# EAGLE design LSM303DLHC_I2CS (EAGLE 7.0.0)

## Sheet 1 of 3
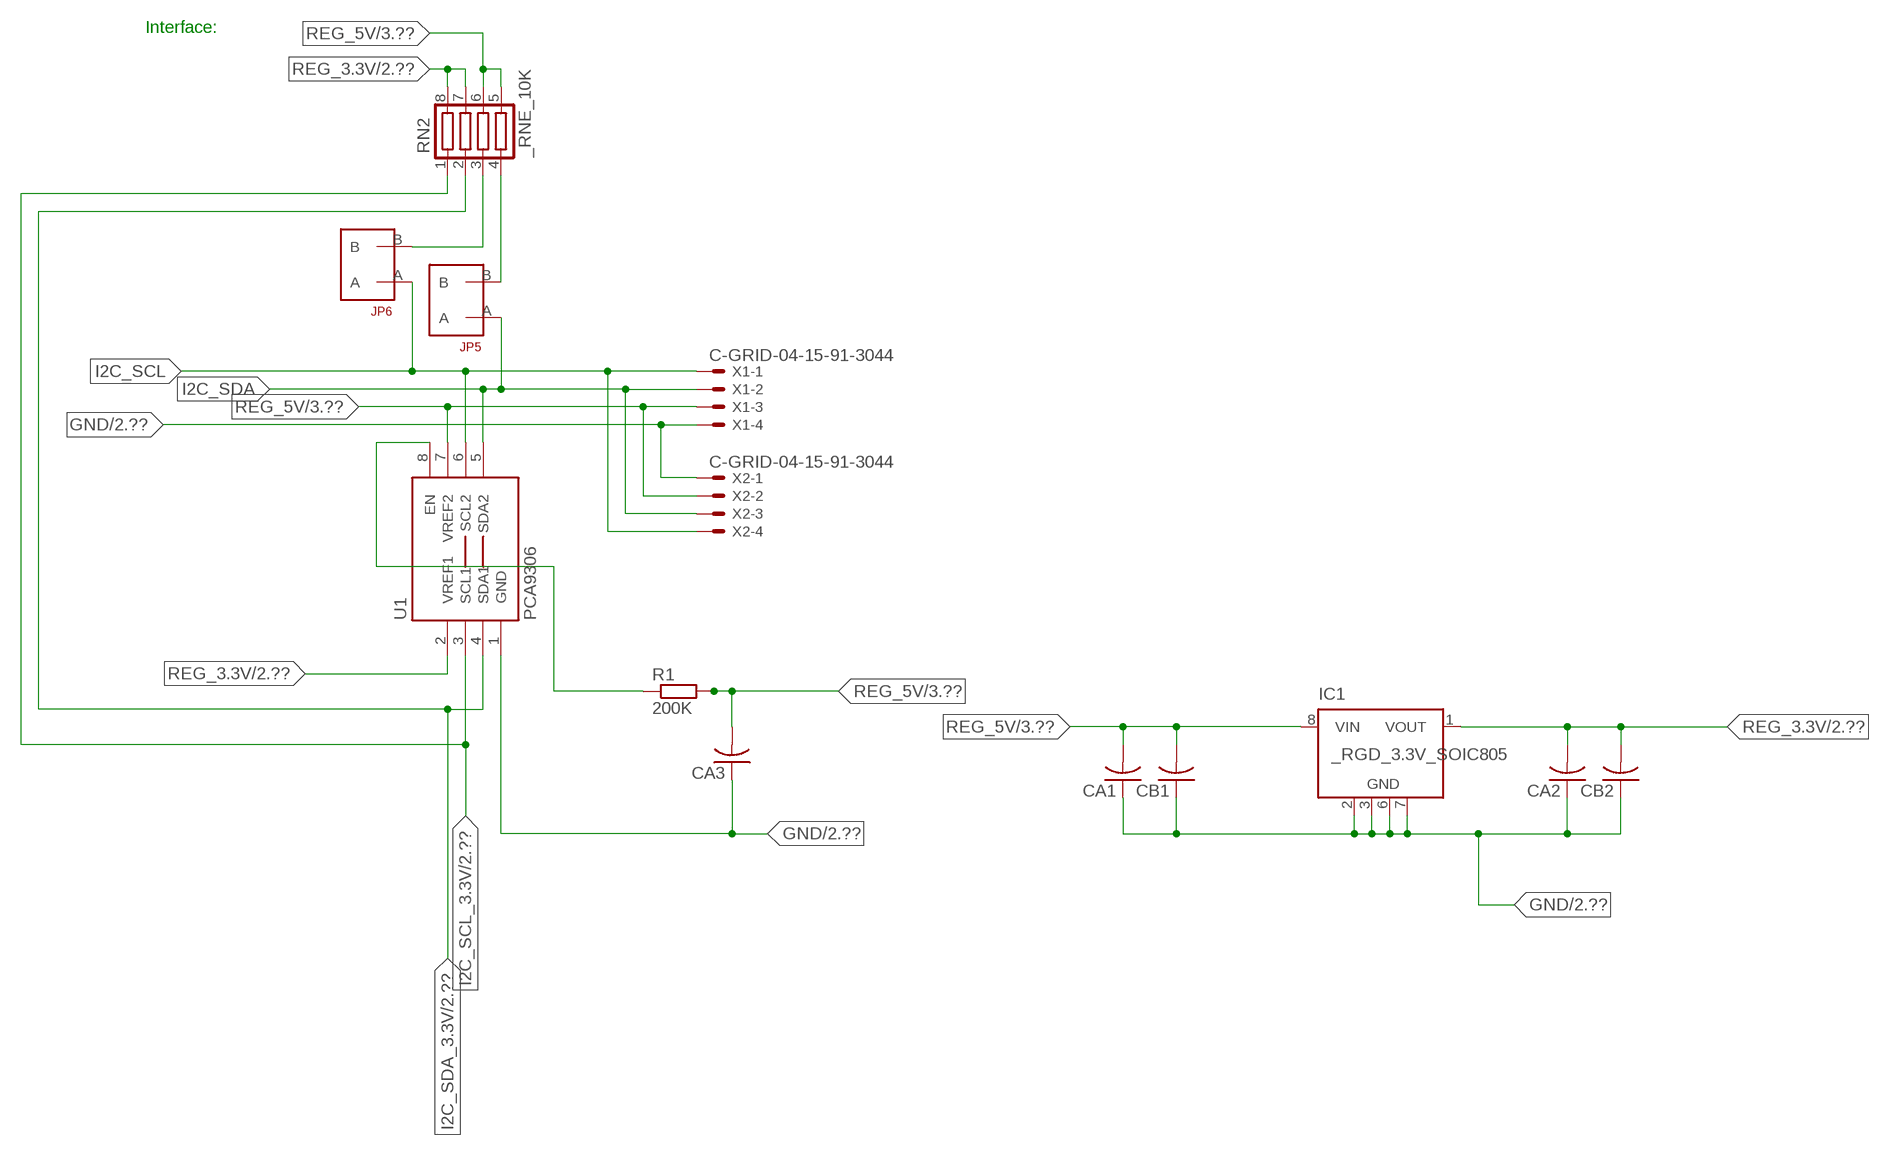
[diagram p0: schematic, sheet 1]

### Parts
CA1  CC1206KRX7R9BB104  [.1UF]
CA2  CC1206KRX7R9BB104  [.1UF]
CA3  CC1206KRX7R9BB104  [.1UF]
CB1  TMK316F106ZL-TC1206K  [TMK316F106ZL-T]
CB2  TMK316F106ZL-TC1206K  [TMK316F106ZL-T]
IC1  _RGD_3.3V_SOIC805  [_RGC_3.3V_SOIC8]
JP5  JUMPER_1X2_2MM  [JUMPER_1X2_2MM]
JP6  JUMPER_1X2_2MM  [JUMPER_1X2_2MM]
R1  200K  RESISTOR_SMT-0603  [R603]
RN2  _RNE_10K  [RNE]
U1  PCA9306  PCA9306_NCD  [PSOP-8]
X1  C-GRID-04-15-91-3044  [15-91-04]
X2  C-GRID-04-15-91-3044  [15-91-04]

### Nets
GND: CA1.1 CA2.1 CA3.1 CB1.1 CB2.1 IC1.2(GND) IC1.3(GND) IC1.6(GND) IC1.7(GND) U1.1(GND) X1.4 X2.1 ; also sheet 2,3
I2C_SCL: JP6.A U1.6(SCL2) X1.1 X2.4
I2C_SCL_3.3V: RN2.1 U1.3(SCL1) ; also sheet 2
I2C_SDA: JP5.A U1.5(SDA2) X1.2 X2.3
I2C_SDA_3.3V: RN2.2 U1.4(SDA1) ; also sheet 2
N$1: JP6.B RN2.3
N$2: JP5.B RN2.4
N$3: R1.1 U1.8(EN)
REG_3.3V: CA2.2 CB2.2 IC1.1(VOUT) RN2.7 RN2.8 U1.2(VREF1) ; also sheet 2
REG_5V: CA1.2 CA3.2 CB1.2 IC1.8(VIN) R1.2 RN2.5 RN2.6 U1.7(VREF2) X1.3 X2.2 ; also sheet 3
Unconnected: IC1.4(NC) IC1.5(NC)

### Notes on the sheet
- Interface:

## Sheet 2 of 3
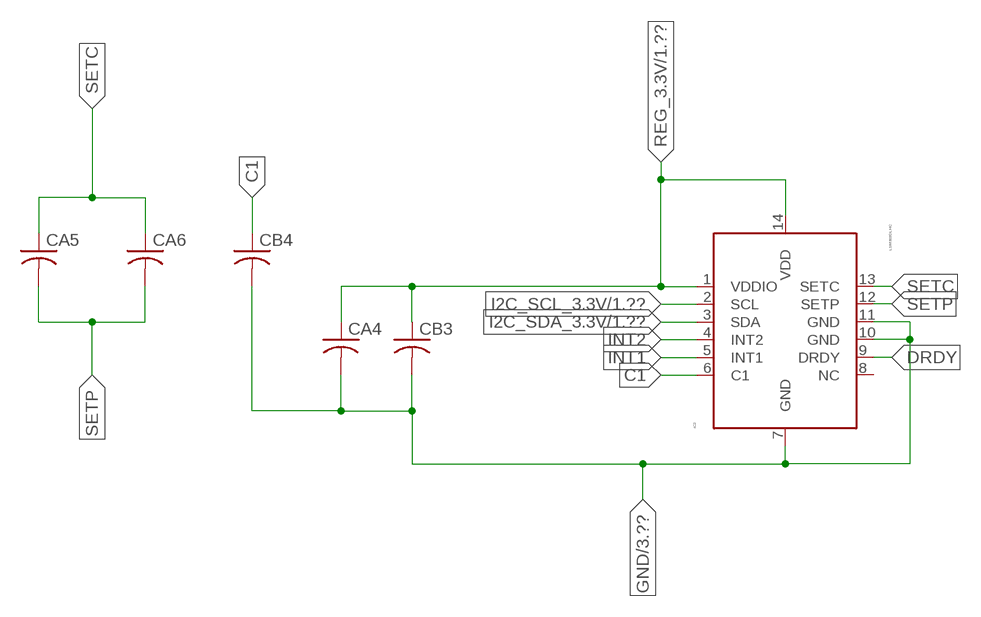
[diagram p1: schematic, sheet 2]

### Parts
CA4  CC1206KRX7R9BB104  [.1UF]
CA5  CC1206KRX7R9BB104  [.1UF]
CA6  CC1206KRX7R9BB104  [.1UF]
CB3  _CB_10UF_25VC1206K  [_CB_10UF_25V]
CB4  _CB_10UF_25VC1206K  [_CB_10UF_25V]
IC2  LSM303DLHC  MICROBUILDER_LSM303DLHC  [MICROBUILDER_LGA14]

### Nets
C1: CB4.1 IC2.6(C1)
DRDY: IC2.9(DRDY)
GND: CA4.2 CB3.2 CB4.2 IC2.7(GND) IC2.10(GND) IC2.11(GND) ; also sheet 1,3
I2C_SCL_3.3V: IC2.2(SCL) ; also sheet 1
I2C_SDA_3.3V: IC2.3(SDA) ; also sheet 1
INT1: IC2.5(INT1)
INT2: IC2.4(INT2)
REG_3.3V: CA4.1 CB3.1 IC2.1(VDDIO) IC2.14(VDD) ; also sheet 1
SETC: CA5.1 CA6.1 IC2.13(SETC)
SETP: CA5.2 CA6.2 IC2.12(SETP)
Unconnected: IC2.8(NC)

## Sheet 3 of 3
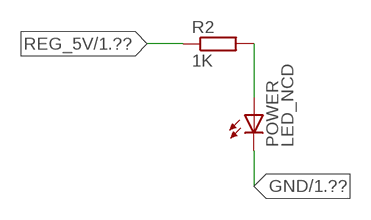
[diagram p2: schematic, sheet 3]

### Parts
POWER  LED_NCD  [CHIPLED_0603]
R2  1K  RESISTOR_SMT-0402  [R402]

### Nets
GND: POWER.C ; also sheet 1,2
N$4: POWER.A R2.2
REG_5V: R2.1 ; also sheet 1

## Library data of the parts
CA1-CA3 = NCD_ULTIMATE_LIBRARY:CC1206KRX7R9BB104: Capacitor CA .1uF 50V SMT C1206K CC1206KRX7R9BB104
CA4-CA6 = NCD_ULTIMATE_LIBRARY (2):CC1206KRX7R9BB104: Capacitor CA .1uF 50V SMT C1206K CC1206KRX7R9BB104
CB1 CB2 = NCD_ULTIMATE_LIBRARY:TMK316F106ZL-T: Capacitor CB 10uF SMT 1206 TMK316F106ZL-T
CB3 CB4 = NCD_ULTIMATE_LIBRARY (2):_CB_10UF_25V: Capacitor 10uF SMT
IC1 = NCD_ULTIMATE_LIBRARY:_RGD_3.3V_SOIC8: Regulator Linear 3.3V Chip Positive VOLTAGE REGULATOR Digikey 497-1199-2-ND/L78L33ACD13TR
IC2 = NCD_ULTIMATE_KAMNA:MICROBUILDER_LSM303DLHC: LSM303DLHC 3-Axis I2C Accelerometer and 3-Axis Magnetometer VDD: 2.2-3.6V VDDIO: 1.8-VDD Magnetic Range: +/-1.3 to +/-8.1 gauss Accel Range: +/-2/4/8/16 g Temp: -40 - 85°C
JP5 JP6 = NCD_ULTIMATE_CONNECTORS:JUMPER_1X2_2MM
POWER = NCD_ULTIMATE_LIBRARY:LED_NCD: LED Digikey 754-1132-2-ND/APT2012SRCPRV
R1 R2 = NCD_ULTIMATE_LIBRARY:RESISTOR_SMT: NCD Resistor
RN2 = NCD_ULTIMATE_LIBRARY:_RNE_10K: Resistor Array RNE SMT 10K x 4 Single Resistor Source: http://www.ctscorp.com/components/Datasheets/CTSChipArrayDs.pdf Digikey 742C083103JPTR-ND/742C083103JP; OC_FARNELL: unknown; OC_NEWARK: unknown
U1 = NCD_ULTIMATE_LIBRARY:PCA9306_NCD: NCD Bidirectional I2C level shifter. NOT compatible with all available part number pinout schemes- DOUBLE CHECK!!!; PROD_ID: IC-10023
X1 X2 = NCD_ULTIMATE_CONNECTORS:C-GRID-04: CONNECTOR 4-Pos I2C wire to board 2.54 mm (0.100") pitch header Digikey WM1342-ND/0015912045; OC_FARNELL: unknown; OC_NEWARK: unknown

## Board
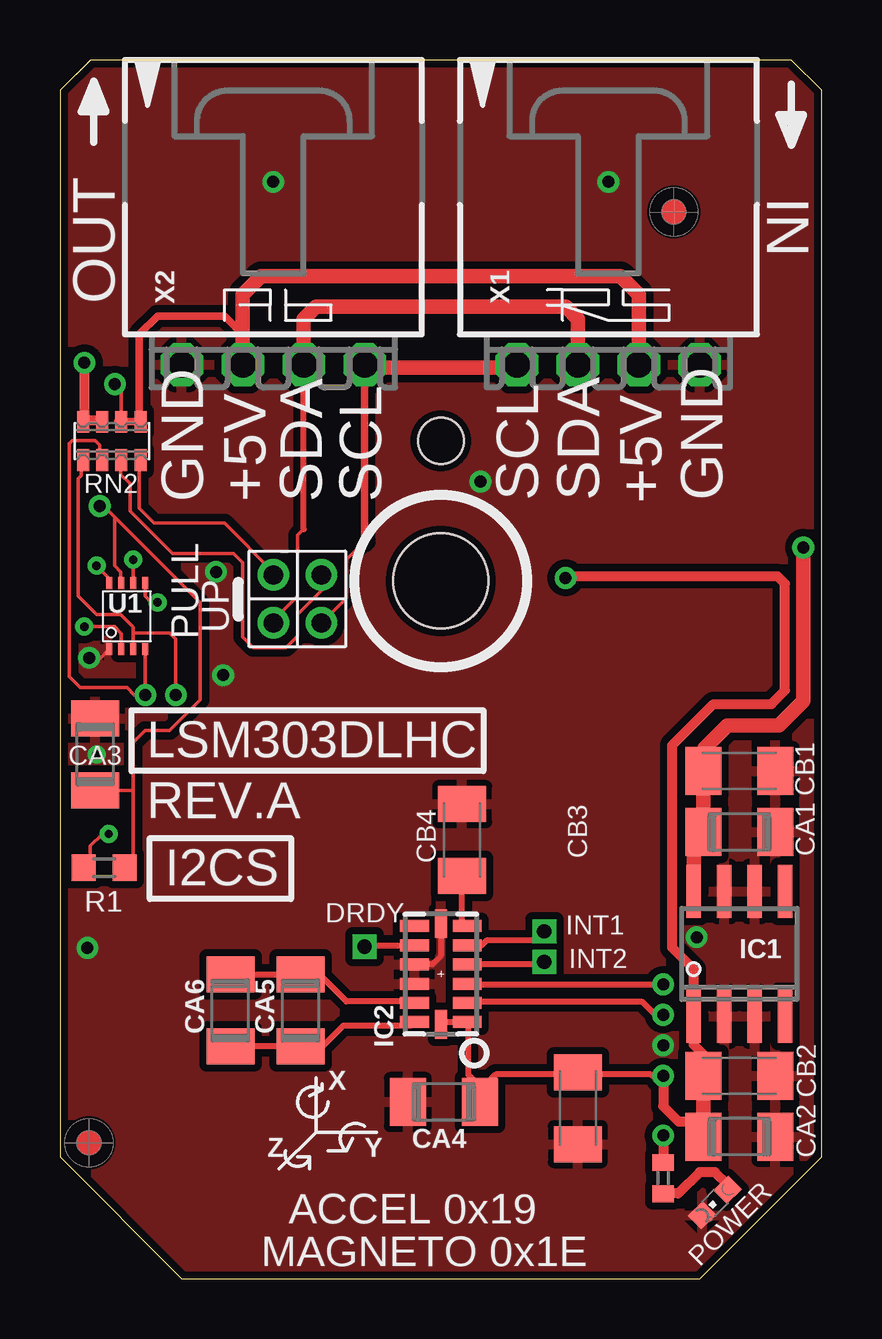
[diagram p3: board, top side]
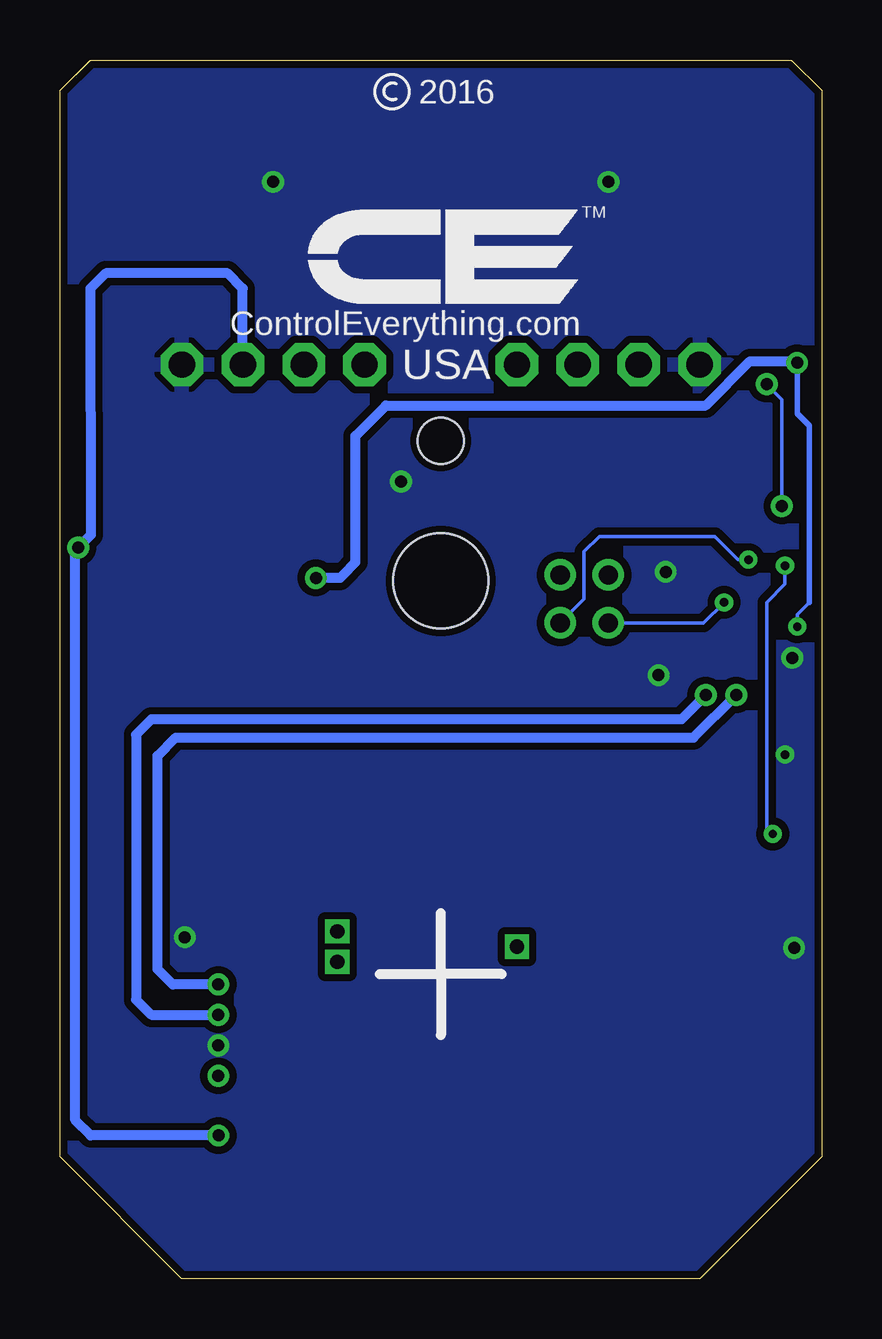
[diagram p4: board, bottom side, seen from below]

Size 31.75 x 50.8 mm. Coordinates in mm from the lower left corner, seen from the top.
Outline: 32 segments
Copper layers (1*16): Top 0.035mm / dielectric 1.5mm / Bottom 0.035mm
Design rules "default": minimum track width 5mil, minimum drill 24mil, track to track 5mil, track to pad 5mil, pad to pad 5mil, via to via 5mil, smd to smd 5mil, copper to edge 10mil, drill to drill 8mil, minimum pad ring 10mil, minimum via ring 8mil, stop-mask expansion 2mil, vias tented up to drill 0mil, thermal gap 10mil
Holes 3.96 mm at 15.88,29.08
Holes 1.91 mm at 15.88,34.93

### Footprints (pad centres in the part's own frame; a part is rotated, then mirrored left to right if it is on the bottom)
.1UF = smd 1.5 x 2: 1 -1.5,0; 2 1.5,0
TMK316F106ZL-T = smd 1.5 x 2: 1 -1.5,0; 2 1.5,0
_CB_10UF_25V = smd 1.5 x 2: 1 -1.5,0; 2 1.5,0
_RGC_3.3V_SOIC8 = smd 0.6 x 2.2: 1 -1.905,-2.6; 2 -0.635,-2.6; 3 0.635,-2.6; 4 1.905,-2.6; 5 1.905,2.6; 6 0.635,2.6; 7 -0.635,2.6; 8 -1.905,2.6
MICROBUILDER_LGA14 = smd 0.5 x 1.2: 1 2,1.1; 2 1.2,1.1; 3 0.4,1.1; 4 -0.4,1.1; 5 -1.2,1.1; 6 -2,1.1; 8 -2,-1.1; 9 -1.2,-1.1; 10 -0.4,-1.1; 11 0.4,-1.1; 12 1.2,-1.1; 13 2,-1.1 | smd 1.2 x 0.5: 7 -2.1,0; 14 2.1,0
JUMPER_1X2_2MM = drill 0.8: A 0,2; B 0,0
CHIPLED_0603 = smd 0.8 x 0.876: A 0,-0.75; C 0,0.75
R603 = smd 1 x 1.1: 1 -0.85,0; 2 0.85,0
R402 = smd 0.7 x 0.9: 1 -0.65,0; 2 0.65,0
RNE = smd 0.5 x 0.9: 1 -1.2,-0.8; 2 -0.4,-0.8; 3 0.4,-0.8; 4 1.2,-0.8; 5 1.2,0.8; 6 0.4,0.8; 7 -0.4,0.8; 8 -1.2,0.8
PSOP-8 = smd 0.25 x 0.5: 1 -0.73,-1.37; 2 -0.23,-1.37; 3 0.27,-1.37; 4 0.77,-1.37; 5 0.77,1.38; 6 0.27,1.38; 7 -0.23,1.38; 8 -0.73,1.38
15-91-04 = drill 1.1 pad 1.778 octagon: 1 -3.81,-7.62; 2 -1.27,-7.62; 3 1.27,-7.62; 4 3.81,-7.62

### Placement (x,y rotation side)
CA1  28.32,18.62 180 top
CA2  28.32,5.92 180 top
CA3  1.46,21.86 270 top
CA4  16,7.37 180 top
CA5  10.03,11.18 90 top
CA6  7.11,11.18 90 top
CB1  28.32,21.16 180 top
CB2  28.32,8.46 180 top
CB3  21.59,7.11 270 top
CB4  16.76,18.29 90 top
IC1  28.32,13.54 0 top
IC2  15.88,12.7 270 top
JP5  8.89,29.34 180 top
JP6  10.9,29.34 180 top
POWER  27.3,3.18 135 top
R1  1.84,17.13 0 top
R2  25.15,4.19 270 top
RN2  2.16,34.93 0 top
U1  2.79,27.61 0 top
U$5  [VISION_REF10]  1.21,5.66 90 top
U$28  [VISION_REF10]  25.59,44.46 90 top
X1  22.86,45.72 0 top
X2  8.89,45.72 0 top

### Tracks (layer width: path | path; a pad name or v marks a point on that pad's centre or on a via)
C1
  Top 0.254: IC2.6 16.76,14.91 CB4.1
DRDY  (via drill 0.6)
  Top 0.254: v12.7,13.84 12.76,13.9 IC2.9
GND  (via drill 0.35, 0.5)
  Top 0.152: CA3.1 1.52,23.42 1.52,23.62 | U1.1 1.7,25.88 v1.22,25.88
  Top 0.254: IC2.7 15.88,13.46 15.51,13.1 IC2.10
  other vias: 8.89,45.72 22.86,45.72 25.15,9.73 6.8,25.16 17.53,33.22 26.55,14.24 1.15,13.79 6.5,29.46 1.52,21.84
  pour Top (isolate 0.305): -1.27,0 -1.27,50.8 33.02,50.8 33.02,0
  pour Bottom (isolate 0.305): -5.08,0 -5.08,50.8 35.56,50.8 35.56,0
I2C_SCL  (via drill 0.35)
  Top 0.152: 12.7,30.73 11.94,29.97 11.94,28.38 JP6.A | v3.05,29.97 3.06,29.96 U1.6
  Top 0.305: 12.7,30.73 X2.4
  Top 0.406: X2.4 12.7,37.97 | 19.05,37.97 X1.1
  Top 0.61: 12.7,37.97 19.05,37.97
  Bottom 0.152: JP6.A 9.91,28.33 9.91,30.3 9.27,30.94 4.45,30.94 3.48,29.97 v3.05,29.97
I2C_SCL_3.3V  (via drill 0.5)
  Top 0.152: RN2.1 0.89,34.07 0.89,33.48 0.77,33.35 0.77,29.1 0.76,29.09 0.76,28.45 1.52,27.69 2.54,27.69 3.06,27.17 3.06,26.92 | 3.06,26.92 U1.3 | v4.83,24.33 v4.83,24.34 4.83,26.67 4.57,26.92 3.06,26.92
  Top 0.254: IC2.2 17.03,11.56 24.26,11.56 24.82,11 v25.15,11
  Bottom 0.406: v4.83,24.33 5.84,23.32 27.94,23.32 28.58,22.68 28.58,11.63 27.94,11 v25.15,11
I2C_SDA  (via drill 0.35)
  Top 0.152: JP5.A 8.89,27.44 9.91,28.45 9.91,30.99 10.16,31.24 | U1.5 3.56,28.45 3.81,28.19 v4.06,28.19
  Top 0.254: 10.16,31.24 10.16,31.25 X2.3
  Top 0.61: X2.3 10.16,40.01 10.67,40.51 21.09,40.51 21.59,40.01 X1.2
  Bottom 0.152: v4.06,28.19 4.92,27.34 JP5.A
I2C_SDA_3.3V  (via drill 0.5)
  Top 0.152: RN2.2 1.65,34.14 1.65,34.75 1.46,34.94 0.51,34.94 0.38,34.81 0.38,26.37 0.38,26.36 0.38,25.1 0.84,24.64 2.79,24.64 3.1,24.33 v3.56,24.33 v3.56,24.34 U1.4
  Top 0.254: IC2.3 17.01,12.27 v25.15,12.27
  Bottom 0.406: v25.15,12.27 27.05,12.27 27.69,12.9 27.69,21.79 26.93,22.56 5.34,22.56 v3.56,24.33
INT1  (via drill 0.6)
  Top 0.254: v20.19,14.48 19.81,14.1 17.78,14.1 17.58,13.9 IC2.5
INT2  (via drill 0.6)
  Top 0.254: v20.19,13.21 20.09,13.1 IC2.4
N$1
  Top 0.152: JP6.B 10.92,29.31 10.92,28.7 9.91,27.69 9.91,26.8 9.42,26.31 8.06,26.31 7.62,26.75 7.62,29.84 7.24,30.23 4.7,30.23 2.92,32 2.92,33.15 2.54,33.53 2.54,34.1 RN2.3
  Top 0.305: 2.54,34.02 RN2.3
N$2
  Top 0.152: JP5.B 8.89,29.46 6.86,31.5 3.94,31.5 3.3,32.13 3.3,34.07 RN2.4
  Top 0.305: 3.37,33.88 RN2.4
N$3  (via drill 0.35)
  Top 0.152: R1.1 1.27,17.41 1.27,18.03 1.78,18.54 v2.03,18.54 | v1.52,29.72 2.06,29.18 U1.8
  Bottom 0.152: v2.03,18.54 2.29,18.8 2.29,28.19 1.52,28.96 v1.52,29.72
N$4
  Top 0.406: POWER.A 27.84,3.92 27.3,4.45 26.67,4.45 25.78,3.56 25.16,3.56 R2.2
REG_3.3V  (via drill 0.35, 0.5)
  Top 0.152: v1.02,27.18 2.29,27.18 2.56,26.9 U1.2
  Top 0.254: IC2.14 15.97,10.7 IC2.1 | IC2.1 17.02,10.66 17.02,8.51 17.4,8.13 CA4.1 17.78,8.13 18.16,8.51 21.59,8.51 | IC2.1 17.01,10.67 | v25.15,8.46 24.69,8.46 24.64,8.51 21.59,8.51 | CB3.1 21.59,8.51
  Top 0.406: CB2.2 26.82,9.35 26.42,9.75 26.42,10.36 | v25.15,8.46 25.15,7.19 25.78,6.55 26.82,6.55 | IC1.1 26.42,12.9 25.53,13.79 25.53,22.24 27.24,23.95 29.66,23.95 30.23,24.52 30.23,28.97 29.91,29.29 21.16,29.29 v21.08,29.21 | 26.52,5.62 CA2.2 | v1.02,38.18 1.02,35.78 | 1.02,35.78 RN2.8 | 1.02,35.78 1.71,35.78 RN2.7
  Top 0.61: CB2.2 26.82,6.55 CA2.2 | 26.42,10.36 IC1.1
  Bottom 0.152: 0.51,28.19 1.02,27.69 v1.02,27.18
  Bottom 0.229: 0.51,28.19 0.51,35.56 1.02,36.07 v1.02,38.18
  Bottom 0.406: v1.02,38.18 1.08,38.24 2.99,38.24 4.83,36.4 18.16,36.4 19.43,35.13 19.43,29.87 19.94,29.34 20.07,29.21 v21.08,29.21
REG_5V  (via drill 0.5)
  Top 0.152: RN2.6 2.56,37.01 v2.29,37.29 | R1.2 3.05,17.49 3.05,20.36 | 3.05,20.36 3.05,22.35 3.56,22.86 4.57,22.86 5.84,24.13 5.84,28.19 2.29,31.75 | CA3.2 3.05,20.36 | 2.29,31.75 1.83,32.21 v1.65,32.21 | U1.7 2.54,29.01 2.54,29.46 2.29,29.72 2.29,31.75
  Top 0.305: 7.62,39.37 7.5,39.37 | 2.42,35.74 RN2.6 RN2.5 3.31,35.8 3.31,39.37 4.07,40.13 6.86,40.13 7.62,39.37 | X2.2 7.62,39.37
  Top 0.406: v25.15,5.97 R2.1
  Top 0.61: X2.2 7.62,41.02 8.38,41.78 23.37,41.78 24.13,41.02 X1.3 | IC1.8 26.42,18.21 CA1.2 CB1.2 26.86,21.2 26.86,22.11 27.82,23.06 29.98,23.06 30.99,24.08 v30.99,30.48
  Bottom 0.152: v1.65,32.21 1.65,36.65 v2.29,37.29
  Bottom 0.406: X1.3 24.13,41.28 24.77,41.91 29.84,41.91 30.48,41.27 30.47,31 v30.99,30.48 31.11,30.36 31.11,6.6 30.48,5.97 v25.15,5.97
SETC
  Top 0.254: IC2.13 14.62,10.54 11.81,10.54 10.95,9.68 CA5.1 CA6.1
SETP
  Top 0.254: CA6.2 CA5.2 10.82,12.68 11.94,11.56 14.58,11.56 14.71,11.43 IC2.12

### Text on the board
tPlace: X | Z | Y
tNames: IN | OUT | GND | +5V | SDA | SCL | SCL | SDA | +5V | GND | PULL | UP | LSM303DLHC | REV.A | CB3 | I2CS | DRDY | INT1 | INT2 | ACCEL 0x19 | MAGNETO 0x1E
bNames: 2016 | TM | ControlEverything.com | USA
